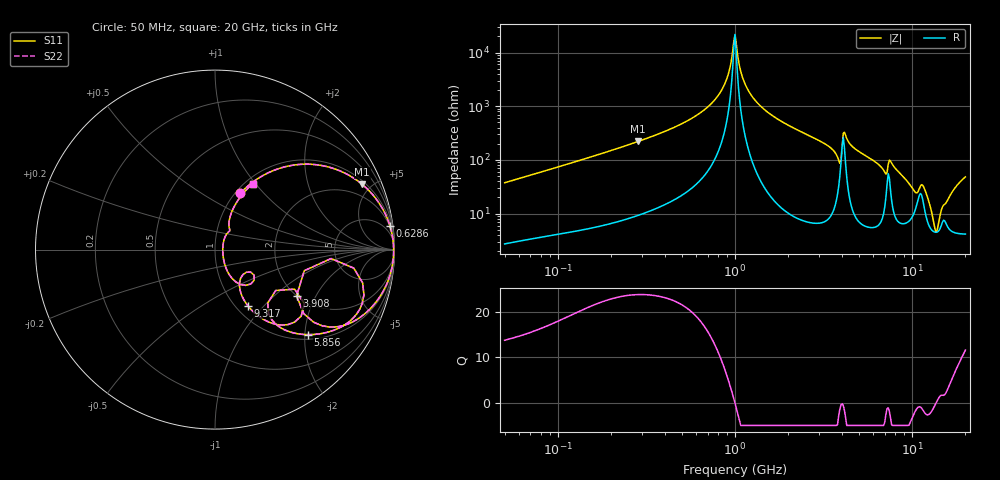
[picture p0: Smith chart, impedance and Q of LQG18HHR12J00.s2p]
!Murata Part Number: LQG18HHR12J00
!These Parameters are Measured in Series Mode Connection
!  o--[Z]--o
!Port1  Port2
!  o-------o
!Freq. Start=50[MHz] Stop=20[GHz], 401[Steps]
# Hz S RI R 50
!Freq.(Hz) S11(Real) S11(Imag) S21(Real) S21(Imag) S12(Real) S12(Imag) S22(Real) S22(Imag)
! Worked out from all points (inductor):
!   401 points, 50 MHz to 20 GHz, reference 50 ohm
!   read as one part in series: L = 118 nH near 51.52 MHz
!   highest Q = 23.8 at 284.2 MHz (marker M1), where L = 124 nH
!   self-resonance near 985.1 MHz
!   S11 on the Smith chart (normalised r, x): 50 MHz: 1.05, +0.75; 628.6 MHz: 2, +15; 3.908 GHz: 1.99, -1.42; 5.856 GHz: 1.11, -2.08; 9.317 GHz: 1.14, -0.82; 20 GHz: 1.08, +0.96
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5e7  0.141 0.3135  0.859 -0.3135  0.859 -0.3135  0.141 0.3135
1.364002e8  0.5041 0.476  0.4959 -0.476  0.4959 -0.476  0.5041 0.476
2.841629e8  0.8202 0.3636  0.1798 -0.3636  0.1798 -0.3636  0.8202 0.3636
3.721004e8  0.8944 0.2867  0.1056 -0.2867  0.1056 -0.2867  0.8944 0.2867
6.285508e8  0.9746 0.1322  0.0254 -0.1322  0.0254 -0.1322  0.9746 0.1322
8.480927e8  0.9925 0.0465  0.0075 -0.0465  0.0075 -0.0465  0.9925 0.0465
1e9  0.9954 -0.000368  0.00458 0.000368  0.00458 0.000368  0.9954 -0.000368
1.127304e9  0.9946 -0.0348  0.00545 0.0348  0.00545 0.0348  0.9946 -0.0348
1.309461e9  0.9897 -0.0788  0.0103 0.0788  0.0103 0.0788  0.9897 -0.0788
2.728004e9  0.8697 -0.3242  0.1303 0.3242  0.1303 0.3242  0.8697 -0.3242
3.626126e9  0.6656 -0.4314  0.3344 0.4314  0.3344 0.4314  0.6656 -0.4314
3.908127e9  0.4545 -0.2584  0.5455 0.2584  0.5455 0.2584  0.4545 -0.2584
4.275624e9  0.8206 -0.2987  0.1794 0.2987  0.1794 0.2987  0.8206 -0.2987
5.856089e9  0.5192 -0.4739  0.4808 0.4739  0.4808 0.4739  0.5192 -0.4739
7.009217e9  0.2983 -0.3561  0.7017 0.3561  0.7017 0.3561  0.2983 -0.3561
7.442007e9  0.4986 -0.3021  0.5014 0.3021  0.5014 0.3021  0.4986 -0.3021
9.316812e9  0.1827 -0.3124  0.8173 0.3124  0.8173 0.3124  0.1827 -0.3124
1.050288e10  0.1429 -0.1591  0.8571 0.1591  0.8571 0.1591  0.1429 -0.1591
1.166392e10  0.1701 -0.1993  0.8299 0.1993  0.8299 0.1993  0.1701 -0.1993
1.375312e10  0.0432 0.00688  0.9568 -0.00688  0.9568 -0.00688  0.0432 0.00688
1.504638e10  0.0821 0.1045  0.9179 -0.1045  0.9179 -0.1045  0.0821 0.1045
2e10  0.2092 0.3658  0.7908 -0.3658  0.7908 -0.3658  0.2092 0.3658
